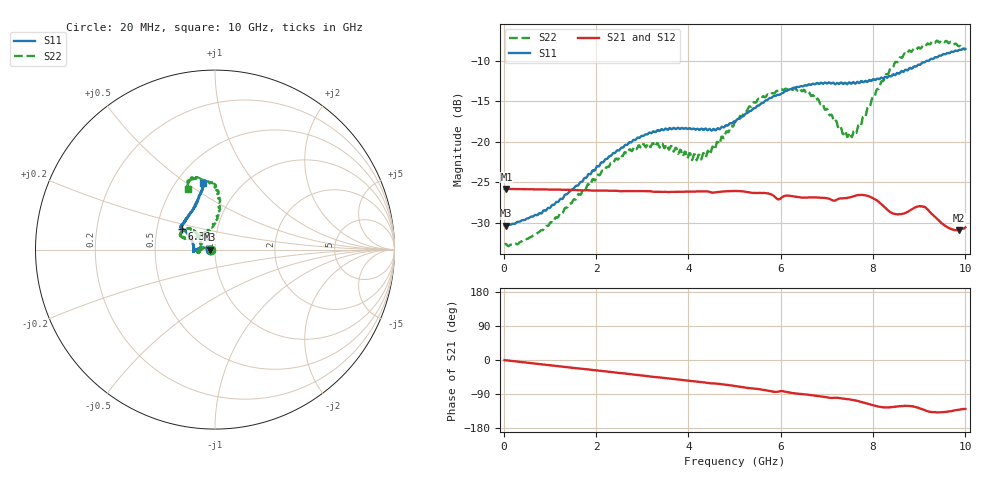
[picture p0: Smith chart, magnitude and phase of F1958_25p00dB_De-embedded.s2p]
! Integrated Device Technology
! Corporate Headquarters
! 6024 Silver Creek Valley Road
! San Jose, CA 95138  USA
! Phone:  1-408-284-8200
! Toll Free:  1-800-223-1366
! Webpage:  http://www.idt.com/
! Timing and RF Division
! 515 Groton Road, Suite 102
! Westford, MA 01886-6024
! Device:  F1958
! Description: 7-bit 0.25 dB Digital Step Attenuator
! Frequency:  0.001 -  6.000 GHz
! Package:  4x4 mm Thin QFN Plastic Package: 24 pin
! Ports:  2 RF, 12 DC
!  Pin  1  = D0
!  Pin  2  = VDD
!  Pin  3  = VMODE
!  Pin  4  = GND
!  Pin  5  = RF1  =  Port 1
!  Pin  6  = GND
!  Pin  7  = GND
!  Pin  8  = GND
!  Pin  9  = GND
!  Pin 10  = GND
!  Pin 11  = GND
!  Pin 12  = GND
!  Pin 13  = GND
!  Pin 14  = RF2  =  Port 2
!  Pin 15  = GND
!  Pin 16  = LE
!  Pin 17  = CLK
!  Pin 18  = DATA
!  Pin 19  = D6
!  Pin 20  = D5
!  Pin 21  = D4
!  Pin 22  = D3
!  Pin 23  = D2
!  Pin 24  = D1
! State:  100
! Atten State:  25.00 dB
! Voltage:  +3.30 Volts
! Current:  0.258 mA
! Data:  The device was measured on a F1958 evaluation board which has
!  individual transmission lines to the RF pins.  Data was collected
!  using a calibrated network analyzer.  The evaluation board was
!  de-embedded using Automatic Fixture Removal (AFR).
!  The reference plane is the edge of the package pin.
! Misc:
!  Action Tracker AT0419
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# GHz S dB R 50
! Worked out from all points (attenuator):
!   500 points, 20 MHz to 10 GHz, reference 50 ohm
!   highest |S21| = -25.83 dB at 60 MHz (marker M1); lowest = -30.9 dB at 9.86 GHz (marker M2)
!   lowest |S11| = -30.4 dB at 40 MHz (marker M3), VSWR 1.06, Z = 47.1 - j0.043 ohm
!   |S11| at or under -10 dB: start of sweep to 9.159 GHz; 9.171289 GHz to 9.203475 GHz (32.19 MHz wide, 0.35 % of centre)
!   |S22| runs from -32.9 to -7.5 dB; largest |S21 - S12| = 0.00036
!   S11 on the Smith chart (normalised r, x): 20 MHz: 0.94, -0.00; 6.36 GHz: 0.67, +0.16; 10 GHz: 0.68, +0.58
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0.02  -30.33 -178.9  -25.83 -0.3  -25.84 -0.3  -32.66 -178.7
0.04  -30.36 -179.1  -25.83 -0.5  -25.83 -0.5  -32.62 -178.3
0.06  -30.35 180.0  -25.83 -0.8  -25.82 -0.8  -32.69 -178.1
0.84  -28.70 171.0  -25.89 -11.6  -25.88 -11.6  -30.92 172.8
1.7  -24.94 171.1  -26.01 -23.2  -25.99 -23.2  -26.10 172.0
2.6  -20.64 177.0  -26.10 -35.3  -26.08 -35.3  -21.53 -179.8
3.36  -18.65 -175.4  -26.18 -45.9  -26.19 -46.0  -20.51 -168.6
4.24  -18.56 -178.8  -26.14 -57.6  -26.15 -57.6  -21.64 169.7
4.5  -18.62 175.3  -26.28 -61.7  -26.29 -61.8  -21.02 152.1
5.02  -17.49 160.9  -26.08 -68.9  -26.09 -68.9  -17.43 138.6
5.58  -15.23 150.6  -26.33 -77.8  -26.35 -77.9  -14.68 140.3
6.36  -13.22 148.1  -26.83 -88.8  -26.85 -88.7  -13.68 155.9
6.68  -12.88 146.7  -26.88 -92.9  -26.90 -92.8  -14.32 158.1
7.5  -12.71 138.4  -26.87 -104.0  -26.88 -104.0  -18.91 120.5
7.68  -12.67 135.5  -26.59 -108.5  -26.59 -108.4  -17.98 100.5
7.9  -12.49 129.1  -26.71 -116.1  -26.71 -116.2  -15.69 89.9
8.34  -11.88 119.1  -28.54 -125.1  -28.55 -125.2  -11.48 84.2
8.66  -11.39 113.4  -28.89 -121.2  -28.89 -121.3  -9.27 87.8
9.1  -10.21 107.2  -28.02 -131.2  -27.98 -131.4  -8.13 100.4
9.58  -9.16 101.1  -30.45 -136.8  -30.45 -137.1  -7.54 109.3
9.86  -8.67 100.0  -30.93 -131.1  -30.94 -131.1  -8.20 112.7
10  -8.54 100.0  -30.59 -129.1  -30.65 -129.1  -8.65 113.9
